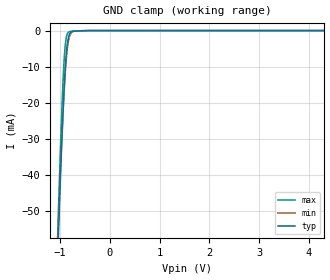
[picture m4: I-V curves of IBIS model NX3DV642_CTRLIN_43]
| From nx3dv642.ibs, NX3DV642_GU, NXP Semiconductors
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|   Model NX3DV642_CTRLIN_43
[Model]   NX3DV642_CTRLIN_43
Model_type   Input
Vinl = 0.7V
Vinh = 1.7V
C_comp   0.852pF   0.806pF   0.911pF
[Model Spec]
| Note: The input and output voltage ratings may be exceeded if the input and
|   output current ratings are observed (please refer to the data sheet)
|   Subparameter   typ   min   max
| Thresholds
Vinl   0.7   0.7   0.7
Vinh   1.7   1.7   1.7
| Overshoot
S_overshoot_high   4.3   4.3   4.3
S_overshoot_low   -0.5   -0.5   -0.5
D_overshoot_high   5.5   5.5   5.5
D_overshoot_low   -0.95   -0.9   -1.0
D_overshoot_time   3n   3n   3n
|Ambient temperature:   25   85   -40
[Temperature Range]   30   90   -35
[Voltage Range]   4.3   4.3   4.3
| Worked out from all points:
|   GND clamp passes 1 mA (typ) near -0.81 V on its own axis
|Process Range   nominal   slow   fast
[GND_clamp]
|   voltage   I(typ)   I(min)   I(max)
-4.3V     -1.553A    -1.422A    -1.69A
-1.062V   -67.87mA   -63.41mA   -61.74mA
-1.047V   -61.37mA   -57.56mA   -54.65mA
-1.031V   -55mA      -51.83mA   -47.72mA
-968.8mV  -31.2mA    -30.51mA   -22.4mA
-921.9mV  -16.31mA   -17.15mA   -8.299mA
-875mV    -6.075mA   -7.52mA    -1.726mA
-843.8mV  -2.534mA   -3.684mA   -580.6uA
-812.5mV  -990.4uA   -1.642mA   -277.3uA
-734.4mV  -207.8uA   -256.9uA   -137.5uA
-437.5mV  -7.087uA   -16.06uA   -2.371uA
4.3V      0A         0A         0A
